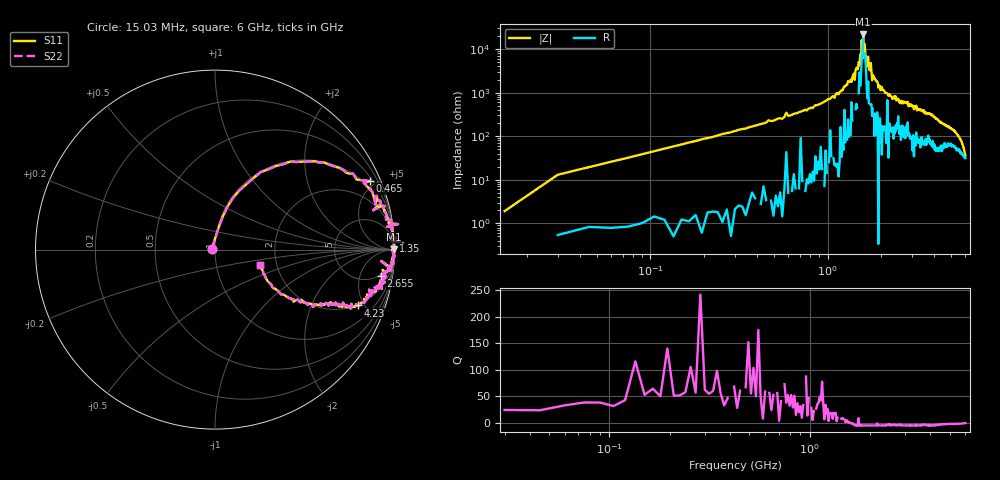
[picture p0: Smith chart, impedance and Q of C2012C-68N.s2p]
!	Network	Analyzer	HP8753E.07.74:	Oct	30	2002	Serial	No.	JP38451487
!	Hewlett-Packard
!	7	Sep	2009	10:58:05
!	Frequency	S11	S21	S12	S22
#	HZ	S	RI	R	50
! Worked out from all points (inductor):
!   400 points, 15.03 MHz to 6 GHz, reference 50 ohm
!   read as one part in series: L = 68.5 nH near 45.03 MHz
!   highest |Z| = 21.7 kohm at 1.59 GHz (marker M1)
!   self-resonance near 1.56 GHz
!   S11 on the Smith chart (normalised r, x): 15.03 MHz: 0.96, +0.01; 465 MHz: 0.68, +4.62; 1.35 GHz: 3, +39; 2.655 GHz: 4, -11; 4.23 GHz: 1.96, -4.47; 6 GHz: 1.63, -0.30
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1.502992e7  -0.0178 0.0044  1.02 -0.0044  1.02 -0.0044  -0.0178 0.0044
3.002985e7  0.0217 0.127  0.978 -0.127  0.978 -0.127  0.0217 0.127
9.002955e7  0.137 0.331  0.863 -0.331  0.863 -0.331  0.137 0.331
4.650277e8  0.861 0.382  0.139 -0.382  0.139 -0.382  0.861 0.382
1.020025e9  0.976 0.136  0.0239 -0.136  0.0239 -0.136  0.976 0.136
1.350023e9  0.995 0.0502  0.00525 -0.0502  0.00525 -0.0502  0.995 0.0502
1.515022e9  0.984 0.0165  0.0157 -0.0165  0.0157 -0.0165  0.984 0.0165
1.560022e9  0.997 0.00555  0.00272 -0.00555  0.00272 -0.00555  0.997 0.00555
1.575022e9  0.984 -0.00174  0.0158 0.00174  0.0158 0.00174  0.984 -0.00174
1.590022e9  0.996 0.00122  0.00443 -0.00122  0.00443 -0.00122  0.996 0.00122
1.605022e9  1 -0.0146  -0.00378 0.0146  -0.00378 0.0146  1 -0.0146
1.620022e9  0.995 -0.00604  0.00467 0.00604  0.00467 0.00604  0.995 -0.00604
1.665022e9  0.992 -0.0236  0.00794 0.0236  0.00794 0.0236  0.992 -0.0236
1.695022e9  0.996 -0.0143  0.00421 0.0143  0.00421 0.0143  0.996 -0.0143
1.785021e9  0.99 -0.0504  0.0103 0.0504  0.0103 0.0504  0.99 -0.0504
2.01002e9  0.985 -0.0736  0.0154 0.0736  0.0154 0.0736  0.985 -0.0736
2.655017e9  0.925 -0.148  0.0751 0.148  0.0751 0.148  0.925 -0.148
3.015015e9  0.946 -0.183  0.0535 0.183  0.0535 0.183  0.946 -0.183
4.00501e9  0.842 -0.283  0.158 0.283  0.158 0.283  0.842 -0.283
4.230009e9  0.794 -0.311  0.206 0.311  0.206 0.311  0.794 -0.311
5.010005e9  0.635 -0.303  0.365 0.303  0.365 0.303  0.635 -0.303
6e9  0.249 -0.0851  0.751 0.0851  0.751 0.0851  0.249 -0.0851
